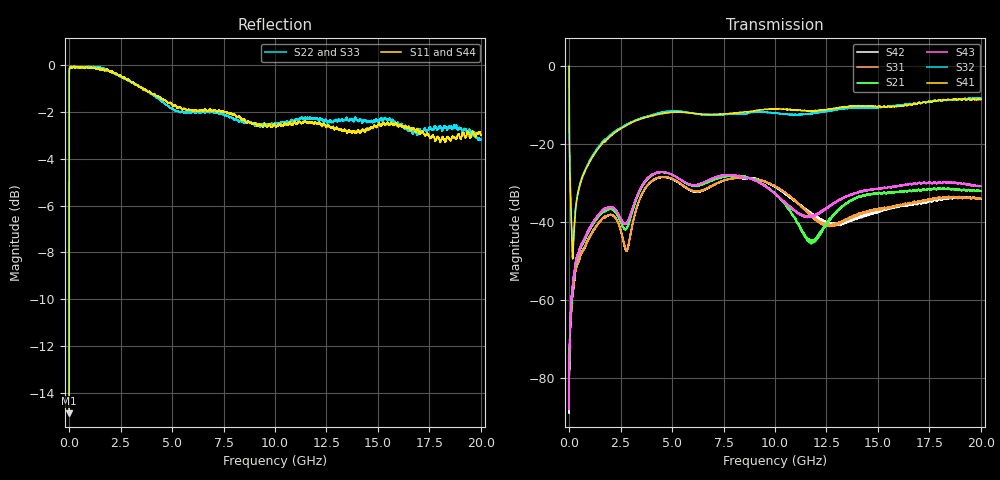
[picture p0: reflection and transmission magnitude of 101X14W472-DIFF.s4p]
!{101X14W472}
!Johanson Technology Inc.
!www.johansontechnology.com
!Test Board Conditions:
!Substrate Type  RO4350B
!Substrate Thickness  10 mil
!Substrate Dk  3.66
!TL Type: GCPW
!TL Trace Width  20 mil
!TL Gap  15 mil
!PART MODE DIFFERENTIAL
!DUT TOPOLOGY	DIFFERENTIAL 4-PORT
!Mounting Pad LxW  20x35 mil
# MHz S  dB  R 50
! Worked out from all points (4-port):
!   20001 points, 300 kHz to 20 GHz, reference 50 ohm
!   strongest paths, dB at 300 kHz, 5 GHz, 10 GHz, 15 GHz, 20 GHz:
!     S41: -0.2, -12.0, -11.1, -10.5, -8.7
!     S32: -0.1, -11.6, -12.2, -10.7, -8.3
!     S43: -82.1, -27.9, -32.8, -31.4, -30.8
!     S21: -86.6, -27.9, -32.7, -32.8, -32.0
!     S31: -82.4, -28.9, -30.8, -36.8, -34.0
!     S42: -74.1, -29.0, -31.0, -37.3, -34.1
!   lowest |S11| = -14.9 dB at 300 kHz (marker M1), VSWR 1.44, Z = 44.2 - j16.3 ohm
!   |S11| at or under -10 dB: start of sweep to 763 kHz
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0.3  -14.87 -99.8  -76.02 56.8  -88.12 -72.7  -0.23 -10.3
     -86.56 -64.5  -14.76 -102.1  -0.18 -10.3  -80.21 102.4
     -82.36 101.3  -0.15 -10.2  -14.80 -101.7  -83.32 -72.9
     -0.23 -10.4  -74.07 74.1  -82.10 109.4  -14.95 -99.5
199.297  -0.08 178.8  -54.90 81.1  -57.33 79.1  -47.20 35.7
         -55.01 79.1  -0.09 178.9  -46.51 39.6  -56.82 78.7
         -56.98 79.5  -46.62 39.6  -0.05 178.8  -54.91 79.0
         -47.13 37.1  -56.77 77.5  -54.92 80.3  -0.16 178.8
1288.281  -0.15 169.5  -39.59 67.2  -41.36 63.5  -22.16 71.9
          -39.57 66.9  -0.07 167.6  -21.80 70.5  -41.42 62.1
          -41.36 63.2  -21.75 70.6  -0.09 167.1  -39.03 66.7
          -22.20 72.0  -41.36 62.6  -39.08 66.6  -0.14 167.2
2801.258  -0.62 159.2  -41.55 67.6  -47.14 57.0  -15.20 51.5
          -41.44 67.6  -0.61 158.3  -15.00 49.2  -47.21 56.5
          -47.29 57.0  -14.98 49.4  -0.66 156.4  -40.19 65.6
          -15.25 51.4  -47.29 55.9  -40.24 65.8  -0.55 157.8
4199.237  -1.29 148.9  -27.58 49.0  -28.93 43.7  -12.62 31.5
          -27.63 49.1  -1.37 151.2  -12.38 30.4  -29.03 43.8
          -28.91 43.6  -12.35 30.3  -1.40 148.3  -27.42 46.8
          -12.63 31.7  -29.01 43.9  -27.45 47.0  -1.37 147.6
11775.12  -2.45 117.6  -45.14 -22.7  -38.64 -89.5  -11.56 -16.7
          -45.38 -22.5  -2.25 118.0  -12.24 -17.4  -37.86 -93.1
          -38.40 -91.1  -12.24 -17.3  -2.21 111.1  -38.45 -17.2
          -11.56 -16.6  -37.99 -91.6  -38.35 -16.0  -2.51 112.4
20000  -3.01 67.9  -32.13 -51.4  -33.94 -98.1  -8.66 -49.7
       -32.01 -51.0  -3.18 70.3  -8.30 -50.2  -33.91 -98.4
       -34.01 -97.8  -8.29 -49.2  -3.15 59.6  -30.78 -55.1
       -8.67 -49.2  -34.05 -97.4  -30.80 -55.6  -2.98 62.1
